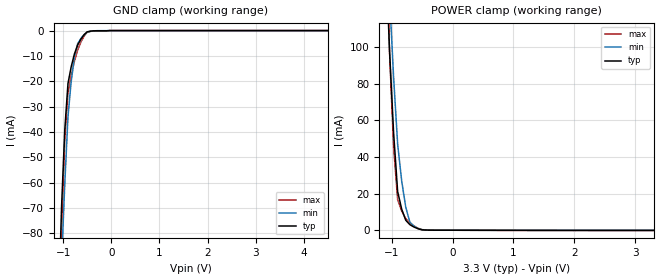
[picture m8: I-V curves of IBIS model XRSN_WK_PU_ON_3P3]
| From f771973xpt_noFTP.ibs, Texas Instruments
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|XRSN_OPEN_DRAIN
|   Model Cell XRSN_WK_PU_ON_3P3
|XRSN_WK_PU_ON_3P3
[Model]   XRSN_WK_PU_ON_3P3
Model_type   Input
Polarity   Non-Inverting
Vinl =  0.8
Vinh =  2
C_comp   4.25494p   0.807076p   4.29559p
[Model Spec]
Vinl   0.8   0.8   0.8
Vinh   2   2   2
[Temperature Range]   25   155   -40
[Voltage Range]   3.3   2.97   3.63
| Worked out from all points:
|   GND clamp passes 1 mA (typ) near -0.53 V on its own axis
|   POWER clamp passes 1 mA (typ) near -0.58 V on its own axis
| Nom Voltages:
|   BIASFET=3.3, VDD=1.2, VDDS=3.3, VSS=0
| Min Voltages:
|   BIASFET=2.97, VDD=1.08, VDDS=2.97, VSS=0
| Max Voltages:
|   BIASFET=3.63, VDD=1.32, VDDS=3.63, VSS=0
[POWER_clamp]
|   voltage   I(typ)   I(min)   I(max)
-3.3V     2.375A     2.63A      3.153A
-1.1V     156mA      180.1mA    173.4mA
-1.033V   98.45mA    128.2mA    97.99mA
-966.7mV  53.5mA     83.9mA     45.75mA
-900mV    21.19mA    47.15mA    16.7mA
-833.3mV  11.49mA    26.82mA    10.5mA
-766.7mV  5.441mA    12.57mA    6.285mA
-700mV    3.052mA    4.404mA    4.065mA
-633.3mV  1.772mA    2.315mA    2.348mA
-500mV    224.9uA    330.4uA    256.9uA
-366.7mV  35.75uA    46.03uA    45.22uA
3.3V      -86.03uA   -56.08uA   -137.9uA
[GND_clamp]
|   voltage   I(typ)   I(min)   I(max)
-3.3V     -1.947A    -1.623A    -3.254A
-1.1V     -112mA     -127.1mA   -135.8mA
-1.033V   -69.63mA   -91.64mA   -80.2mA
-966.7mV  -39.25mA   -60.63mA   -43.14mA
-900mV    -20.89mA   -34.03mA   -24.56mA
-833.3mV  -14.31mA   -20.13mA   -17.7mA
-766.7mV  -9.259mA   -10.54mA   -12.12mA
-700mV    -5.75mA    -5.235mA   -7.84mA
-566.7mV  -1.652mA   -1.611mA   -2.192mA
-500mV    -488.4uA   -625.8uA   -598.3uA
-33.33mV  0A         0A         0A
6.6V      0A         0A         0A
